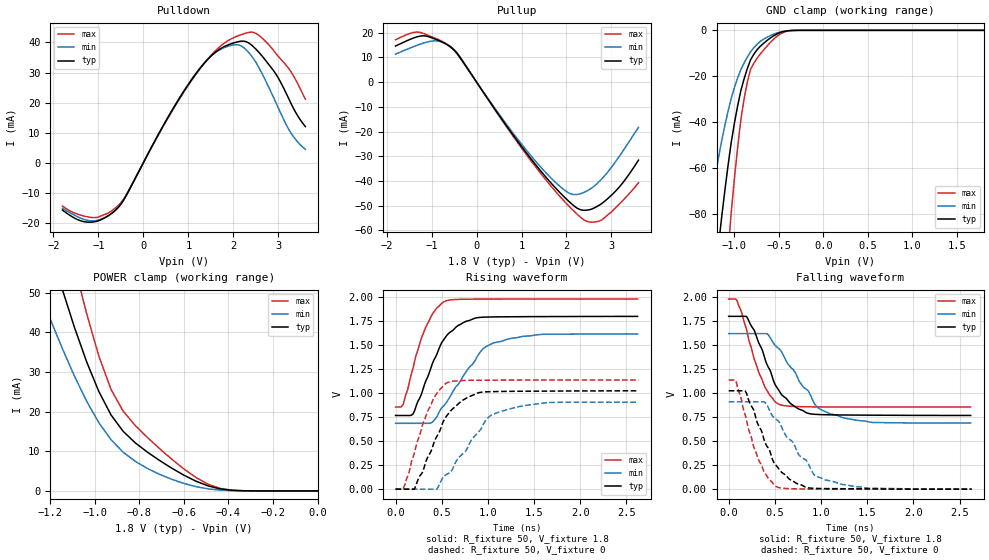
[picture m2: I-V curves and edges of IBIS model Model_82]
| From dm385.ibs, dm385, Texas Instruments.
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| Model based on original model for BCSHTLTCSCDVPBFZ_SSDHV
|   Sub model SR11_10MA_10PER_1P8
[model]   Model_82
|[Description]  [1.8V-3-STATE-NOTERM-SLOWEST:10MA, IND, 10%]
|   Slowest slew rate (SR[1:0] = "11"), 0.80 * RExt = 1.250 * Iout
|   (I[2:0] = "101"), 10mA nominal with Rext = 50R,ODT off (ODT[1:0]
|   = "00") CMOS mode,Industrial temperature range (-40C to 125C,
|   25C nominal),10% power supply tolerance
|[Input Load]   NOTERM
|[Output Drive] SLOWEST:10MA
|Voltage   1.8V
|Mode   3-STATE
Model_type   3-state
Polarity   Non-Inverting
Enable   Active-Low
Cref =  15pF
Rref =  100.0000M
Vref =  0V
Vmeas =  0.9
C_comp   1.851324p   1.663768p   1.973575p
[Temperature Range]   25   125   -40
[Voltage Range]   1.8   1.62   1.98
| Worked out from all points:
|   slope of the pulldown table from 0 to 0.27 V, typ, clamps not added: 35.3 ohm
|   slope of the pullup table from 0 to 0.27 V, typ, clamps not added: 36.9 ohm
|   GND clamp passes 1 mA (typ) near -0.49 V on its own axis
|   POWER clamp passes 1 mA (typ) near -0.47 V on its own axis
|   rising waveform, R_fixture 50, V_fixture 1.8: 20-80 % time 275ps typ, 394ps min, 222ps max; typ from 0.767 V to 1.8 V
|   rising waveform, R_fixture 50, V_fixture 0: 20-80 % time 298ps typ, 386ps min, 237ps max; typ from 0 V to 1.02 V
|   falling waveform, R_fixture 50, V_fixture 1.8: 20-80 % time 285ps typ, 368ps min, 222ps max; typ from 1.8 V to 0.767 V
|   falling waveform, R_fixture 50, V_fixture 0: 20-80 % time 275ps typ, 392ps min, 221ps max; typ from 1.02 V to 0 V
[POWER_clamp]
-1.8V     194.9mA    137.1mA    262.8mA
-1.236V   68.49mA    48.51mA    92.67mA
-1.145V   50.76mA    35.86mA    69.65mA
-1.127V   47.56mA    33.54mA    65.34mA
-1.055V   35.4mA     24.69mA    48.69mA
-981.8mV  25.06mA    17.2mA     34.01mA
-927.3mV  19.17mA    12.93mA    25.61mA
-872.7mV  15.03mA    9.767mA    20.12mA
-818.2mV  12.12mA    7.45mA     16.5mA
-654.5mV  5.738mA    2.93mA     8.003mA
-436.4mV  508.2uA    199.4uA    613uA
0V        2.273nA    15.95nA    16.67nA
[Pulldown]
-1.8V     -15.77mA   -15.17mA   -14.43mA
-1.145V   -19.78mA   -19.39mA   -18.25mA
-545.5mV  -14.66mA   -14.65mA   -14.05mA
545.5mV   15.06mA    15.08mA    14.82mA
1.091V    28.02mA    28.13mA    27.77mA
1.527V    35.81mA    35.8mA     36.1mA
1.964V    39.64mA    39.08mA    41.28mA
2.291V    40.23mA    37.46mA    43.16mA
2.618V    35.85mA    30.21mA    41.73mA
2.945V    29.48mA    19.99mA    36.31mA
3.218V    21.69mA    11.43mA    31.57mA
3.6V      12mA       4.465mA    21.1mA
[Pullup]
-1.8V     14.55mA    11.29mA    17.09mA
-1.2V     18.67mA    15.62mA    19.77mA
-872.7mV  17.03mA    16.61mA    17.36mA
-600mV    14.45mA    14.5mA     14.65mA
-381.8mV  10.35mA    10.1mA     10.52mA
1.2V      -30.78mA   -29.58mA   -31.57mA
1.745V    -42.59mA   -40.36mA   -43.98mA
2.127V    -49.46mA   -45.37mA   -51.49mA
2.455V    -51.78mA   -44mA      -56.34mA
2.727V    -49.78mA   -40.23mA   -56.19mA
3.164V    -42.65mA   -30.28mA   -49.49mA
3.6V      -31.58mA   -18.34mA   -40.72mA
[GND_clamp]
-1.8V     -346.1mA   -209.3mA   -568.3mA
-1.327V   -149.7mA   -89.03mA   -250.9mA
-1.291V   -135.6mA   -80.47mA   -227.5mA
-1.145V   -82.35mA   -48.67mA   -137.7mA
-1.073V   -59.44mA   -35.55mA   -97.96mA
-1.036V   -49.1mA    -29.72mA   -79.9mA
-927.3mV  -26.31mA   -17.11mA   -38.99mA
-854.5mV  -16.67mA   -11.64mA   -22.56mA
-818.2mV  -12.86mA   -9.351mA   -16.98mA
-672.7mV  -5.705mA   -3.913mA   -8.624mA
-381.8mV  -120.4uA   -129uA     -167.4uA
1.8V      2.273nA    454nA      6.646nA
[Ramp]
dV/dt_f 0.62213184/0.28413445n 0.56325916/0.37125251n 0.67638917/0.22199219n
dV/dt_r 0.61758669/0.29768016n 0.54938571/0.38712261n   0.683717/0.2371722n
R_load = 50
[Rising Waveform]
R_fixture = 50
V_fixture = 1.8
V_fixture_min = 1.62
V_fixture_max = 1.98
0s        767.5mV    685.8mV    856mV
82.4ps    767.5mV    685.8mV    881.3mV
192.2ps   789mV      685.8mV    1.271V
330.9ps   1.135V     685.8mV    1.697V
527.3ps   1.564V     874.2mV    1.954V
765.3ps   1.749V     1.226V     1.978V
951.5ps   1.791V     1.466V     1.98V
1.062ns   1.794V     1.524V     1.98V
1.591ns   1.797V     1.613V     1.98V
2.62ns    1.799V     1.617V     1.98V
[Rising Waveform]
R_fixture = 50
V_fixture = 0
V_fixture_min = 0
V_fixture_max = 0
0s        0V         0V         0V
82.4ps    0V         0V         0V
202.8ps   0V         0V         374mV
349.4ps   336.7mV    0V         814.9mV
443.8ps   544.1mV    0V         992.4mV
554.9ps   765.2mV    155.1mV    1.107V
780.3ps   955.7mV    433.5mV    1.133V
1.054ns   1.016V     779.3mV    1.135V
1.654ns   1.021V     902.4mV    1.137V
2.63ns    1.024V     905.5mV    1.137V
[Falling Waveform]
R_fixture = 50
V_fixture = 1.8
V_fixture_min = 1.62
V_fixture_max = 1.98
0s        1.799V     1.619V     1.979V
90.9ps    1.799V     1.619V     1.959V
196.6ps   1.793V     1.619V     1.649V
388.3ps   1.371V     1.619V     1.072V
552ps     1.015V     1.455V     880.4mV
751.7ps   837.5mV    1.15V      859.7mV
941.2ps   778.7mV    871.5mV    856.4mV
1.102ns   773.6mV    783.1mV    855.5mV
1.558ns   770.2mV    694.2mV    855mV
2.62ns    767.3mV    688.7mV    855mV
[Falling Waveform]
R_fixture = 50
V_fixture = 0
V_fixture_min = 0
V_fixture_max = 0
0s        1.024V     909.6mV    1.136V
81.9ps    1.024V     909.6mV    1.115V
179.7ps   1.021V     909.6mV    770.7mV
327.1ps   654.6mV    909.6mV    298.3mV
515.6ps   245.5mV    725.2mV    26.56mV
732.4ps   61.01mV    409.3mV    3.247mV
924ps     8.711mV    150.4mV    0V
1.039ns   6.243mV    97.98mV    0V
1.503ns   3.306mV    11mV       0V
2.63ns    0V         3.159mV    0V
